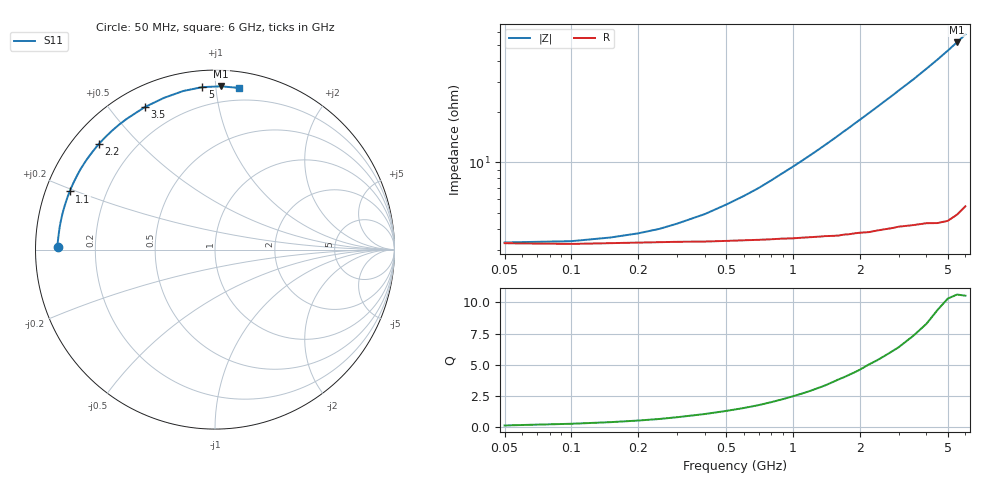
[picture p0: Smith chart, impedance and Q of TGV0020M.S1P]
! SIEMENS Discrete & RF Semiconductors
! BAT64
! Si Schottky Diode in SOT23
! IF = 20 mA
! S-Parameters:  February  1997
# GHz  S  MA  R  50
!  f  S11
! GHz  MAG  ANG
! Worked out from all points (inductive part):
!   34 points, 50 MHz to 6 GHz, reference 50 ohm
!   read as one part to ground: L = 1.38 nH near 1.3 GHz
!   highest Q = 10.5 at 5.5 GHz (marker M1), where L = 1.5 nH
!   S11 on the Smith chart (normalised r, x): 50 MHz: 0.07, +0.01; 1.1 GHz: 0.07, +0.19; 2.2 GHz: 0.08, +0.38; 3.5 GHz: 0.08, +0.62; 5 GHz: 0.09, +0.92; 6 GHz: 0.11, +1.15
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0.05  0.8766 178.9
0.1  0.8778 177.9
0.25  0.8752 174.9
0.4  0.8745 171.8
0.5  0.8738 169.8
0.6  0.8732 167.9
0.7  0.8729 166.0
0.8  0.8725 164.0
0.9  0.872 162.0
1  0.8723 160.1
1.1  0.872 158.2
1.3  0.872 154.4
1.5  0.8726 150.6
1.6  0.8731 148.7
1.7  0.8727 146.8
1.8  0.8731 145.0
1.9  0.873 143.1
2.2  0.875 137.7
2.4  0.8753 134.2
2.6  0.8764 130.7
2.8  0.8777 127.4
3  0.879 124.0
3.5  0.8852 116.2
4  0.892 108.5
4.5  0.9012 101.3
5  0.9079 94.4
5.5  0.9104 87.8
6  0.9105 81.7
